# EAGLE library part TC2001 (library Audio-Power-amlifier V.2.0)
TRIPATH TECHNOLOGY
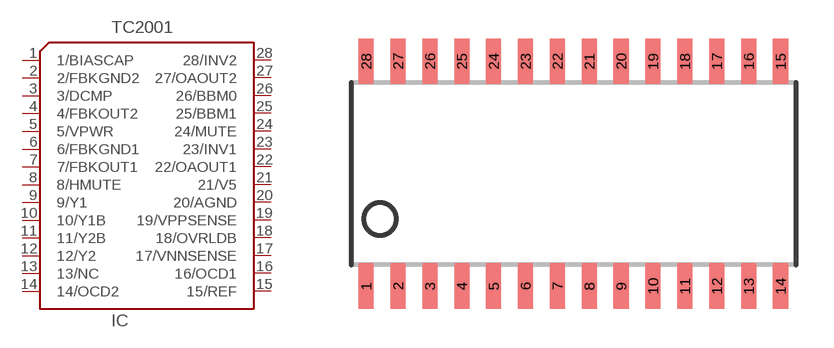
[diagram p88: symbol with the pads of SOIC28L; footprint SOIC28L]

Designator prefix IC

## TC2001  [SOIC28L]
1  1/BIASCAP
2  2/FBKGND2  pwr
3  3/DCMP
4  4/FBKOUT2  out
5  5/VPWR  pwr
6  6/FBKGND1  pwr
7  7/FBKOUT1  out
8  8/HMUTE
9  9/Y1
10  10/Y1B
11  11/Y2B
12  12/Y2
13  13/NC  nc
14  14/OCD2
15  15/REF
16  16/OCD1
17  17/VNNSENSE
18  18/OVRLDB
19  19/VPPSENSE
20  20/AGND  pwr
21  21/V5  pwr
22  22/OAOUT1  out
23  23/INV1  in
24  24/MUTE
25  25/BBM1
26  26/BBM0
27  27/OAOUT2  pwr
28  28/INV2  in

## Footprint SOIC28L (pad centres in mm)
SMALL OUTLINE PACKAGE 17.9 x 10.3
smd 0.6 x 1.8: 1 -8.255,-4.475; 2 -6.985,-4.475; 3 -5.715,-4.475; 4 -4.445,-4.475; 5 -3.175,-4.475; 6 -1.905,-4.475; 7 -0.635,-4.475; 8 0.635,-4.475; 9 1.905,-4.475; 10 3.175,-4.475; 11 4.445,-4.475; 12 5.715,-4.475; 13 6.985,-4.475; 14 8.255,-4.475; 15 8.255,4.475; 16 6.985,4.475; 17 5.715,4.475; 18 4.445,4.475; 19 3.175,4.475; 20 1.905,4.475; 21 0.635,4.475; 22 -0.635,4.475; 23 -1.905,4.475; 24 -3.175,4.475; 25 -4.445,4.475; 26 -5.715,4.475; 27 -6.985,4.475; 28 -8.255,4.475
